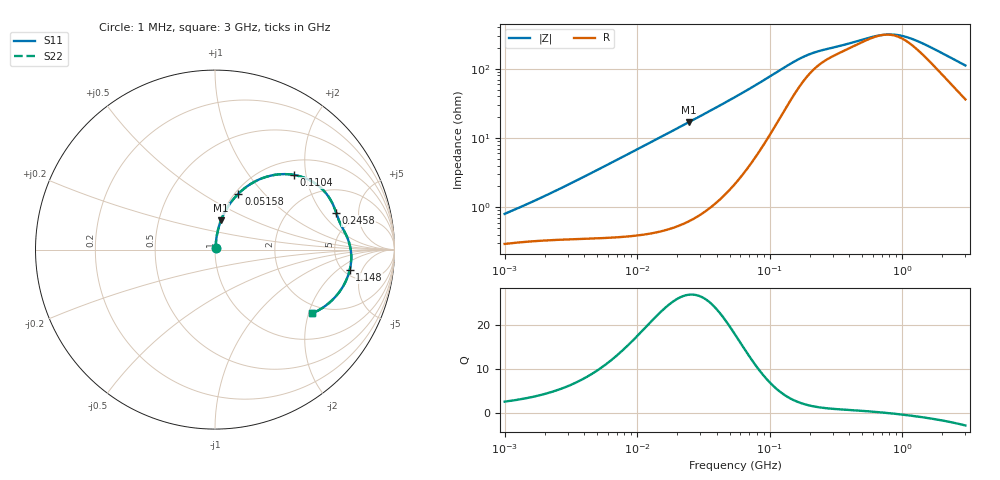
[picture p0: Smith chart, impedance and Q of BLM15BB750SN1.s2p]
! BLM15BB750SN1
# Hz S RI R 50
!Freq.(Hz) S11(Real) S11(Imag) S21(Real) S21(Imag) S12(Real) S12(Imag) S22(Real) S22(Imag)
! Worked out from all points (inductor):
!   401 points, 1 MHz to 3 GHz, reference 50 ohm
!   read as one part in series: L = 114 nH near 1.297 MHz
!   highest Q = 27 at 24.6 MHz (marker M1), where L = 110 nH
!   self-resonance near 730.6 MHz
!   S11 on the Smith chart (normalised r, x): 1 MHz: 1.01, +0.01; 51.58 MHz: 1.04, +0.73; 110.4 MHz: 1.30, +1.71; 245.8 MHz: 3.42, +2.78; 1.148 GHz: 5.61, -3.04; 3 GHz: 1.72, -2.11
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1000000  0.003 0.00742  0.997 -0.00742  0.997 -0.00742  0.003 0.00742
1786863  0.00342 0.0126  0.9966 -0.0126  0.9966 -0.0126  0.00342 0.0126
3823119  0.00417 0.0262  0.9958 -0.0262  0.9958 -0.0262  0.00417 0.0262
8017732  0.00671 0.0544  0.9933 -0.0544  0.9933 -0.0544  0.00671 0.0544
1.461624e7  0.0142 0.0983  0.9858 -0.0983  0.9858 -0.0983  0.0142 0.0983
2.459509e7  0.0336 0.1627  0.9664 -0.1627  0.9664 -0.1627  0.0336 0.1627
3.670325e7  0.0697 0.2352  0.9303 -0.2352  0.9303 -0.2352  0.0697 0.2352
5.15801e7  0.1305 0.3116  0.8695 -0.3116  0.8695 -0.3116  0.1305 0.3116
5.477226e7  0.1455 0.3258  0.8545 -0.3258  0.8545 -0.3258  0.1455 0.3258
6.690963e7  0.2075 0.371  0.7925 -0.371  0.7925 -0.371  0.2075 0.371
8.173662e7  0.2892 0.4065  0.7108 -0.4065  0.7108 -0.4065  0.2892 0.4065
1.103592e8  0.4397 0.4161  0.5603 -0.4161  0.5603 -0.4161  0.4397 0.4161
1.295243e8  0.5194 0.3911  0.4806 -0.3911  0.4806 -0.3911  0.5194 0.3911
1.550909e8  0.5925 0.3416  0.4075 -0.3416  0.4075 -0.3416  0.5925 0.3416
2.094008e8  0.6597 0.2459  0.3403 -0.2459  0.3403 -0.2459  0.6597 0.2459
2.457655e8  0.6757 0.2041  0.3243 -0.2041  0.3243 -0.2041  0.6757 0.2041
6.049187e8  0.7463 0.0416  0.2537 -0.0416  0.2537 -0.0416  0.7463 0.0416
8.005644e8  0.7584 -0.0217  0.2416 0.0217  0.2416 0.0217  0.7584 -0.0217
9.585869e8  0.7582 -0.0669  0.2418 0.0669  0.2418 0.0669  0.7582 -0.0669
1.147801e9  0.7504 -0.1148  0.2496 0.1148  0.2496 0.1148  0.7504 -0.1148
1.855641e9  0.6842 -0.2473  0.3158 0.2473  0.3158 0.2473  0.6842 -0.2473
3e9  0.5412 -0.3557  0.4588 0.3557  0.4588 0.3557  0.5412 -0.3557
